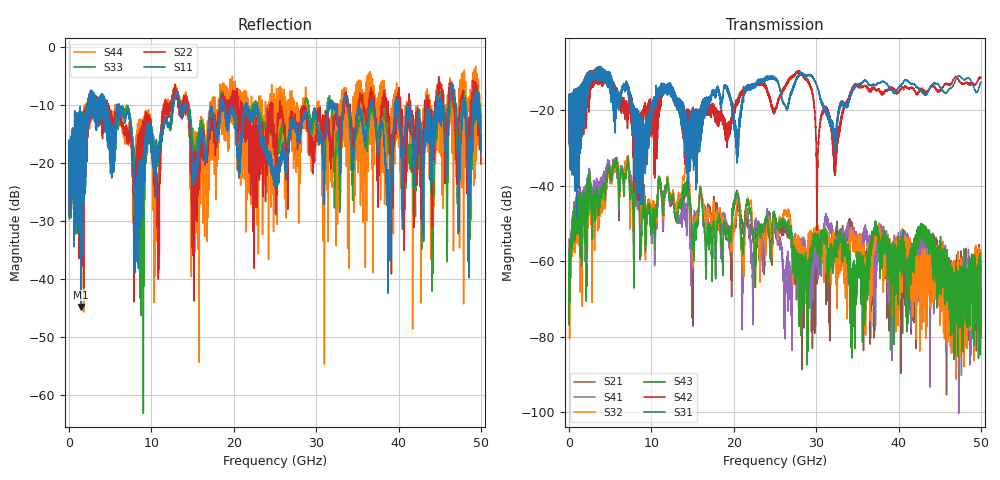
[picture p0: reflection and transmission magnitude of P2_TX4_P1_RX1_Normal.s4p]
!Keysight Technologies,N5225B,MY57041031,A.13.20.10
!Date: Friday, May 31, 2019 11:14:49
!Correction: S11(Full 4 Port(1,2,3,4))
!S12(Full 4 Port(1,2,3,4))
!S13(Full 4 Port(1,2,3,4))
!S14(Full 4 Port(1,2,3,4))
!S21(Full 4 Port(1,2,3,4))
!S22(Full 4 Port(1,2,3,4))
!S23(Full 4 Port(1,2,3,4))
!S24(Full 4 Port(1,2,3,4))
!S31(Full 4 Port(1,2,3,4))
!S32(Full 4 Port(1,2,3,4))
!S33(Full 4 Port(1,2,3,4))
!S34(Full 4 Port(1,2,3,4))
!S41(Full 4 Port(1,2,3,4))
!S42(Full 4 Port(1,2,3,4))
!S43(Full 4 Port(1,2,3,4))
!S44(Full 4 Port(1,2,3,4))
!S4P File: Measurements: <S11,S12,S13,S14>,
!<S21,S22,S23,S24>,
!<S31,S32,S33,S34>,
!<S41,S42,S43,S44>:
# Hz S  dB  R 50.0
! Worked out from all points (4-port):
!   5000 points, 10 MHz to 50 GHz, reference 50 ohm
!   strongest paths, dB at 10 MHz, 12.51 GHz, 25.01 GHz, 37.51 GHz, 50 GHz:
!     S31: -19.2, -14.2, -11.3, -12.8, -12.5
!     S42: -19.5, -14.7, -19.9, -14.6, -11.3
!     S43: -56.8, -44.0, -48.8, -54.0, -67.2
!     S32: -69.8, -43.4, -48.5, -50.9, -65.6
!     S41: -67.8, -43.8, -50.7, -53.9, -64.2
!     S21: -54.1, -44.9, -51.1, -53.5, -60.8
!   lowest |S11| = -44.9 dB at 1.43 GHz (marker M1), VSWR 1.01, Z = 49.4 + j0.131 ohm
!   |S11| at or under -10 dB: 6.023 GHz to 12.61 GHz (6.592 GHz wide, 70.7 % of centre); 14.2 GHz to 18.43 GHz (4.229 GHz wide, 25.9 % of centre); 22.71 GHz to 31.52 GHz (8.805 GHz wide, 32.5 % of centre)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
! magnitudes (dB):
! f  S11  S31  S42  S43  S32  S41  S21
! 10 MHz  -19.0  -19.2  -19.5  -56.8  -69.8  -67.8  -54.1
! 1.43 GHz  -44.9  -26.9  -26.6  -47.4  -47.9  -45.7  -46.3
! 7.02 GHz  -11.4  -12.6  -19.9  -34.8  -32.9  -35.6  -34.8
! 8.18 GHz  -30.1  -21.0  -30.5  -41.8  -38.9  -45.1  -40.4
! 27.85 GHz  -15.7  -11.0  -9.6  -61.8  -55.1  -59.4  -59.5
! 32.27 GHz  -10.9  -27.0  -31.6  -55.1  -55.3  -53.4  -57.3
! 50 GHz  -15.0  -12.5  -11.3  -67.2  -65.6  -64.2  -60.8
